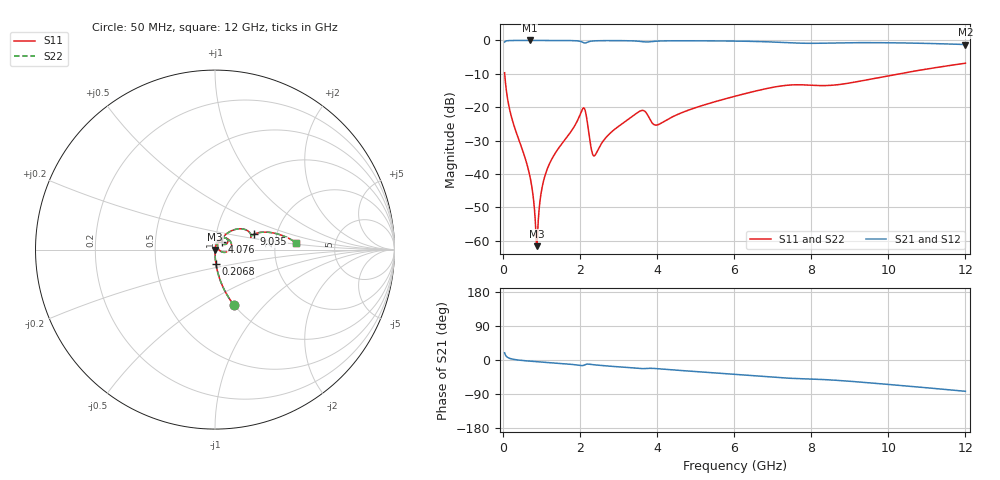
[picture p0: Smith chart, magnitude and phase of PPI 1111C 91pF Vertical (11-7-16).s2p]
# GHz S MA R 50
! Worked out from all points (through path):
!   1601 points, 50 MHz to 12 GHz, reference 50 ohm
!   highest |S21| = -0.01 dB at 699.8 MHz (marker M1); lowest = -1.2 dB at 12 GHz (marker M2)
!   group delay of S21, straight-line fit = 18.9 ps
!   lowest |S11| = -61.7 dB at 886.5 MHz (marker M3), VSWR 1.00, Z = 50.1 + j0.00917 ohm
!   |S11| at or under -10 dB: 52.14 MHz to 10.28 GHz (10.23 GHz wide, 198 % of centre)
!   |S22| runs from -61.7 to -6.8 dB; largest |S21 - S12| = 0
!   S11 on the Smith chart (normalised r, x): 50 MHz: 1.00, -0.69; 206.8 MHz: 1.00, -0.16; 4.076 GHz: 1.07, +0.09; 9.035 GHz: 1.52, +0.27; 12 GHz: 2.65, +0.25
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0.05  0.328 -71.1  0.9444 18.9  0.9444 18.9  0.328 -71.1
0.2068437  0.07949 -86.2  0.9964 3.5  0.9964 3.5  0.07949 -86.2
0.6997813  0.009562 -88.7  0.9992 -3.0  0.9992 -3.0  0.009562 -88.7
0.7744688  0.005439 -85.7  0.9992 -3.6  0.9992 -3.6  0.005439 -85.7
0.8491562  0.001803 -68.2  0.9992 -4.2  0.9992 -4.2  0.001803 -68.2
0.8865  0.0008262 6.4  0.9991 -4.5  0.9991 -4.5  0.0008262 6.4
0.9238437  0.002051 61.3  0.9991 -4.8  0.9991 -4.8  0.002051 61.3
1.020938  0.006208 76.2  0.999 -5.5  0.999 -5.5  0.006208 76.2
1.162844  0.01212 78.7  0.9989 -6.6  0.9989 -6.6  0.01212 78.7
2.044156  0.08711 47.3  0.956 -14.7  0.956 -14.7  0.08711 47.3
2.14125  0.08846 4.7  0.9149 -12.3  0.9149 -12.3  0.08846 4.7
2.298094  0.02368 -6.4  0.9763 -11.7  0.9763 -11.7  0.02368 -6.4
2.372781  0.01865 25.5  0.9851 -12.6  0.9851 -12.6  0.01865 25.5
2.783562  0.04055 66.0  0.9936 -16.3  0.9936 -16.3  0.04055 66.0
3.560313  0.0873 48.7  0.9684 -22.6  0.9684 -22.6  0.0873 48.7
4.038312  0.05482 45.6  0.9786 -23.1  0.9786 -23.1  0.05482 45.6
4.075656  0.05611 48.2  0.9806 -23.4  0.9806 -23.4  0.05611 48.2
6.025  0.1459 47.5  0.9778 -38.1  0.9778 -38.1  0.1459 47.5
8.019156  0.2128 19.2  0.9049 -50.3  0.9049 -50.3  0.2128 19.2
9.034906  0.2322 21.5  0.9244 -56.4  0.9244 -56.4  0.2322 21.5
10.01331  0.2965 19.2  0.9229 -64.6  0.9229 -64.6  0.2965 19.2
12  0.4554 4.7  0.868 -82.6  0.868 -82.6  0.4554 4.7
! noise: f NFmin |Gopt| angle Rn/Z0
0.05  0.0003531  0.8594  0.4825  0.0005376
1.372  0.004089  0.6968  6.865  0.002626
2.701  0.01215  0.7899  13.55  0.01175
4.031  0.02762  0.8588  20.12  0.04058
5.36  0.01915  0.7499  26.28  0.01464
6.682  0.03683  0.834  32.57  0.04321
8.012  0.07469  0.901  38.7  0.1471
9.341  0.05902  0.8614  44.4  0.07832
10.67  0.05015  0.8237  49.73  0.04926
12  0.04836  0.8041  54.76  0.04056
